(* Logix 5000 Routine export Unit1_Shutdown; software revision 20.05 *)

TYPE Unit_Type :   // Common information for a unit
STRUCT
   Alm_Reset : BOOL;   // Alarm reset
   Local : BOOL;   // Local/remote control indication
   Maint : BOOL;   // Maintenance privilege for device control
   Man_StartOpen : BOOL;   // Manual start/open from operator
   Man_StopClose : BOOL;   // Manual stop/close from operator
   Man_DevNum : DINT;   // Number of device started/stopped at OI
   Msg : DINT;   // Message number
   Time_Remaining : DINT;   // Remaining time in timed steps
END_STRUCT
END_TYPE

TYPE Seq_Type :   // Sequence Information
STRUCT
   Step_Num : DINT;   // Current step number
   Running : BOOL;   // Running indication
   PC_Start : BOOL;   // Sequence start request from PC
   LTP_Start : BOOL;   // Sequence start request from LTP
   Ons : BOOL;   // One-shot storage to start
   Auto_Start : BOOL;   // Auto-start request
   Auto_Ons : BOOL;   // Auto-start one-shot storage
   Req_Tmr : TIMER;   // Auto-start hold timer
END_STRUCT
END_TYPE

VAR_GLOBAL   (* controller tags *)
   Unit1_Hold : Seq_Type := (Req_Tmr.PRE := 5000);   // Unit Desc1 Hold Sequence
   Unit1_Sample : Seq_Type := (Req_Tmr.PRE := 5000);   // Unit Desc1 Sample Sequence
   Unit1 : Unit_Type;   // Unit Desc1
   Unit1_Shutdown : Seq_Type := (Req_Tmr.PRE := 5000);   // Unit Desc1 Shutdown Sequence
   Unit1_Eshutdown : Seq_Type := (Req_Tmr.PRE := 5000);   // Unit Desc1 E-Shutdown Sequence
END_VAR

PROGRAM MainProgram

ROUTINE Unit1_Shutdown   (* ladder *)
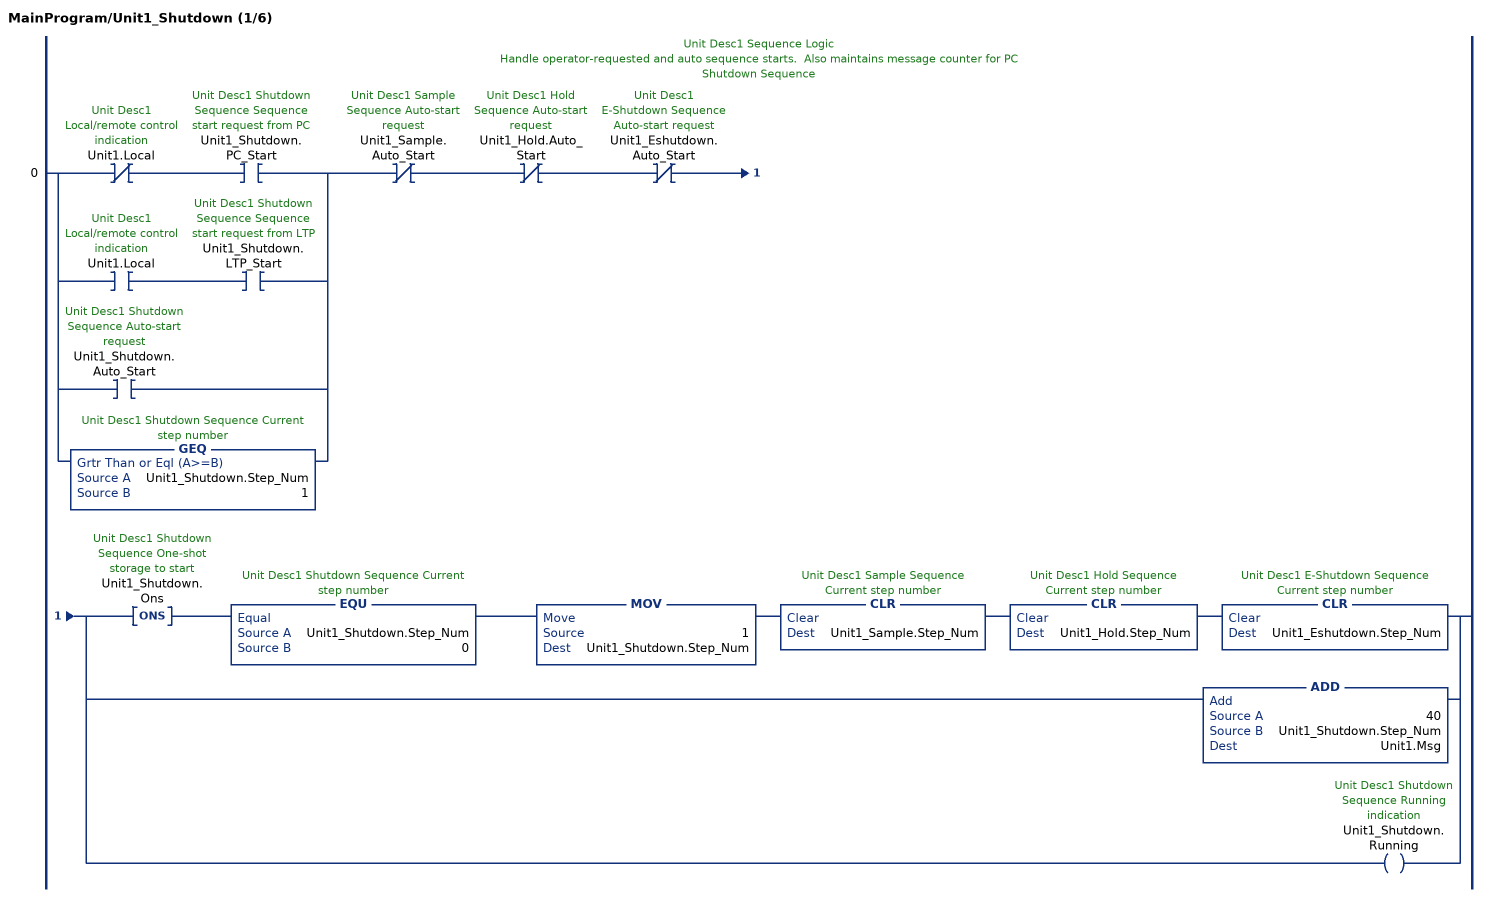
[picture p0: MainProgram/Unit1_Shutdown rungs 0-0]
   // Unit Desc1 Sequence Logic
   // Handle operator-requested and auto sequence starts.  Also maintains message counter for PC
   // Shutdown Sequence
   0: [XIO(Unit1.Local) XIC(Unit1_Shutdown.PC_Start) ,XIC(Unit1.Local) XIC(Unit1_Shutdown.LTP_Start) ,XIC(Unit1_Shutdown.Auto_Start) ,GEQ(Unit1_Shutdown.Step_Num,1) ]XIO(Unit1_Sample.Auto_Start)XIO(Unit1_Hold.Auto_Start)XIO(Unit1_Eshutdown.Auto_Start)[ONS(Unit1_Shutdown.Ons) EQU(Unit1_Shutdown.Step_Num,0) MOV(1,Unit1_Shutdown.Step_Num) CLR(Unit1_Sample.Step_Num) CLR(Unit1_Hold.Step_Num) CLR(Unit1_Eshutdown.Step_Num) ,ADD(40,Unit1_Shutdown.Step_Num,Unit1.Msg) ,OTE(Unit1_Shutdown.Running) ];
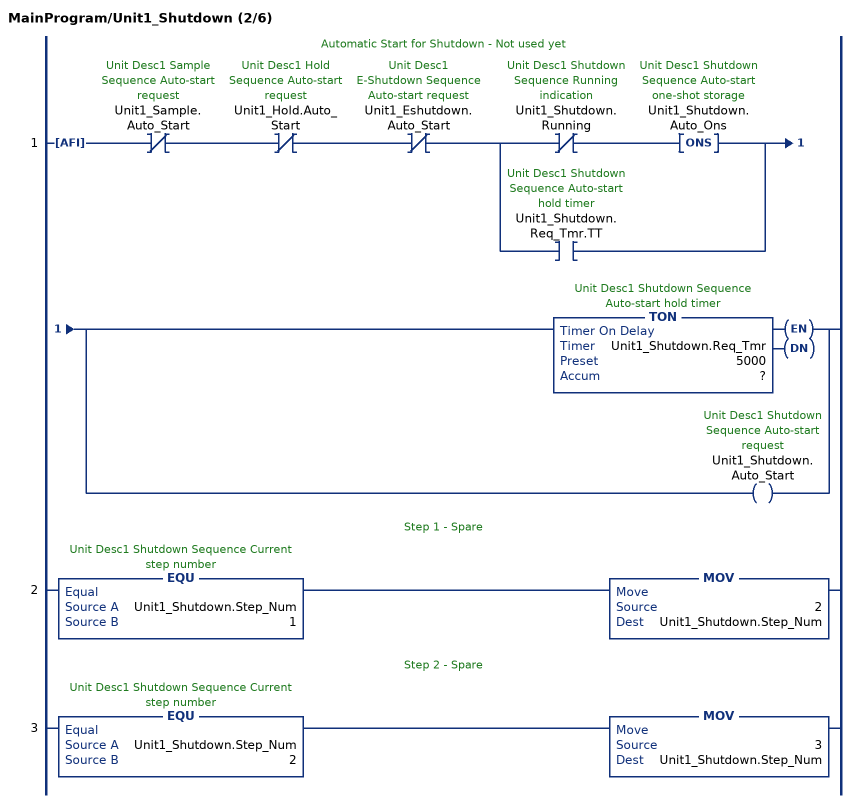
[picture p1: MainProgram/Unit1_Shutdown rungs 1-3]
   // Automatic Start for Shutdown - Not used yet
   1: AFI()XIO(Unit1_Sample.Auto_Start)XIO(Unit1_Hold.Auto_Start)XIO(Unit1_Eshutdown.Auto_Start)[XIO(Unit1_Shutdown.Running) ONS(Unit1_Shutdown.Auto_Ons) ,XIC(Unit1_Shutdown.Req_Tmr.TT) ][TON(Unit1_Shutdown.Req_Tmr,?,?) ,OTE(Unit1_Shutdown.Auto_Start) ];
   // Step 1 - Spare
   2: EQU(Unit1_Shutdown.Step_Num,1)MOV(2,Unit1_Shutdown.Step_Num);
   // Step 2 - Spare
   3: EQU(Unit1_Shutdown.Step_Num,2)MOV(3,Unit1_Shutdown.Step_Num);
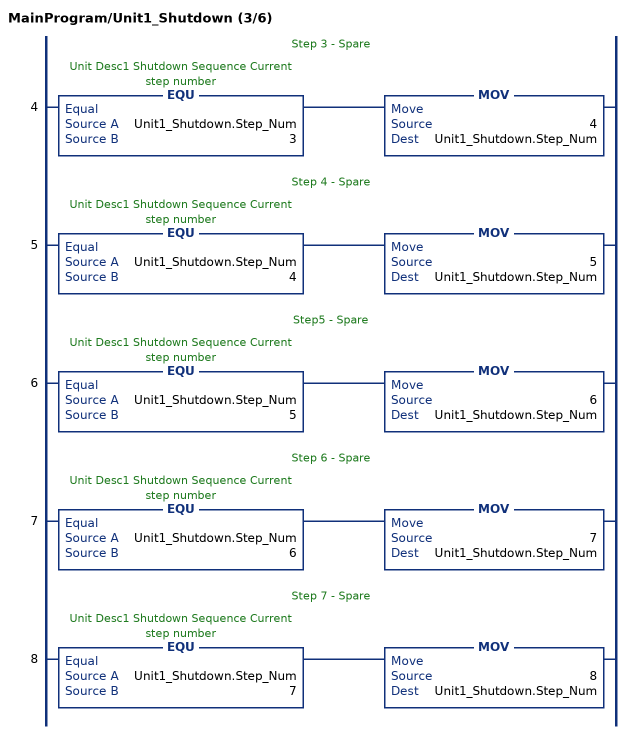
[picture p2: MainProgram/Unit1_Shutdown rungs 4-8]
   // Step 3 - Spare
   4: EQU(Unit1_Shutdown.Step_Num,3)MOV(4,Unit1_Shutdown.Step_Num);
   // Step 4 - Spare
   5: EQU(Unit1_Shutdown.Step_Num,4)MOV(5,Unit1_Shutdown.Step_Num);
   // Step5 - Spare
   6: EQU(Unit1_Shutdown.Step_Num,5)MOV(6,Unit1_Shutdown.Step_Num);
   // Step 6 - Spare
   7: EQU(Unit1_Shutdown.Step_Num,6)MOV(7,Unit1_Shutdown.Step_Num);
   // Step 7 - Spare
   8: EQU(Unit1_Shutdown.Step_Num,7)MOV(8,Unit1_Shutdown.Step_Num);
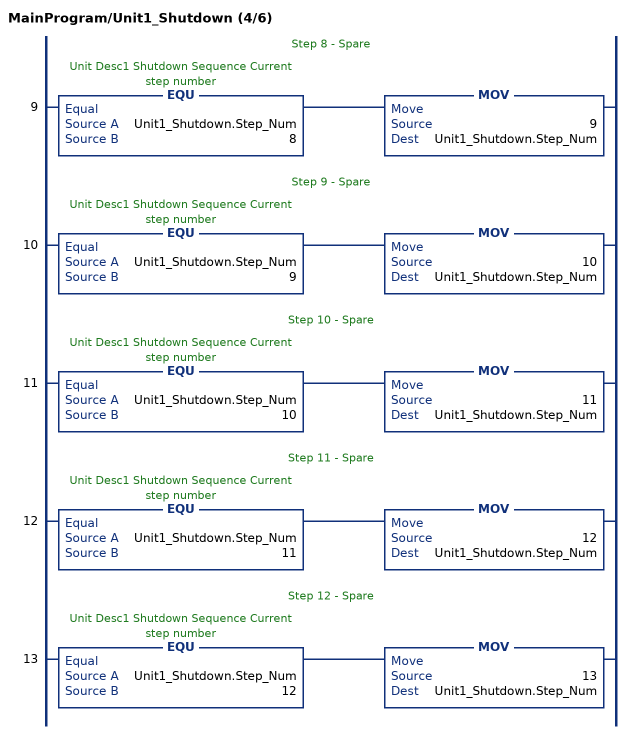
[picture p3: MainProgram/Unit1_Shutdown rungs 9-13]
   // Step 8 - Spare
   9: EQU(Unit1_Shutdown.Step_Num,8)MOV(9,Unit1_Shutdown.Step_Num);
   // Step 9 - Spare
   10: EQU(Unit1_Shutdown.Step_Num,9)MOV(10,Unit1_Shutdown.Step_Num);
   // Step 10 - Spare
   11: EQU(Unit1_Shutdown.Step_Num,10)MOV(11,Unit1_Shutdown.Step_Num);
   // Step 11 - Spare
   12: EQU(Unit1_Shutdown.Step_Num,11)MOV(12,Unit1_Shutdown.Step_Num);
   // Step 12 - Spare
   13: EQU(Unit1_Shutdown.Step_Num,12)MOV(13,Unit1_Shutdown.Step_Num);
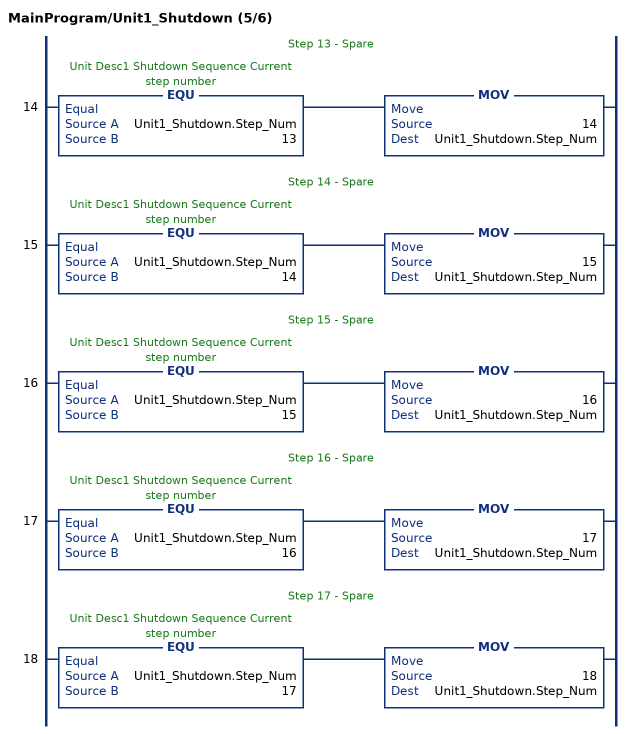
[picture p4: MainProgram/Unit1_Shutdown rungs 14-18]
   // Step 13 - Spare
   14: EQU(Unit1_Shutdown.Step_Num,13)MOV(14,Unit1_Shutdown.Step_Num);
   // Step 14 - Spare
   15: EQU(Unit1_Shutdown.Step_Num,14)MOV(15,Unit1_Shutdown.Step_Num);
   // Step 15 - Spare
   16: EQU(Unit1_Shutdown.Step_Num,15)MOV(16,Unit1_Shutdown.Step_Num);
   // Step 16 - Spare
   17: EQU(Unit1_Shutdown.Step_Num,16)MOV(17,Unit1_Shutdown.Step_Num);
   // Step 17 - Spare
   18: EQU(Unit1_Shutdown.Step_Num,17)MOV(18,Unit1_Shutdown.Step_Num);
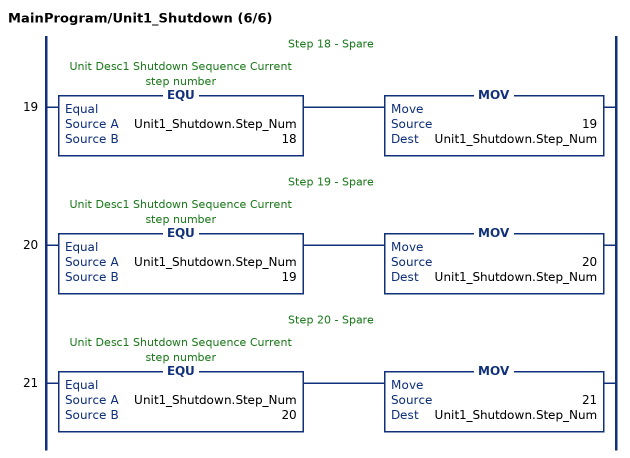
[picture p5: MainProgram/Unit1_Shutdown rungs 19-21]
   // Step 18 - Spare
   19: EQU(Unit1_Shutdown.Step_Num,18)MOV(19,Unit1_Shutdown.Step_Num);
   // Step 19 - Spare
   20: EQU(Unit1_Shutdown.Step_Num,19)MOV(20,Unit1_Shutdown.Step_Num);
   // Step 20 - Spare
   21: EQU(Unit1_Shutdown.Step_Num,20)MOV(21,Unit1_Shutdown.Step_Num);
END_ROUTINE
END_PROGRAM
